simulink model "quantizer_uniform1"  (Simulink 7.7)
settings: Solver=FixedStepDiscrete  StartTime=0.0  StopTime=10  FixedStep=1/fs  RelTol=1e-3
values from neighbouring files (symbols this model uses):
  k = sqrt(10^(atenuation/10))    [quantizer_test.m]
undefined symbols (not defined in the file or in its folder): fs
libraries: dspquant2 x1, dspsrcs4 x1

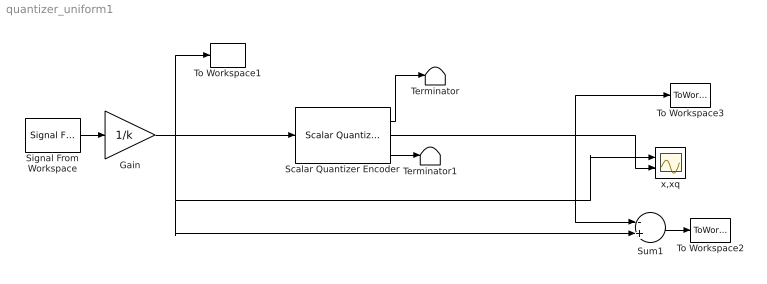
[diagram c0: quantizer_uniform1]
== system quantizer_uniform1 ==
  Gain : Gain  Gain=1/k
  Scalar Quantizer Encoder : dspquant2/Scalar Quantizer Encoder  paramSrc=Specify via dialog  partType=Bounded  BBoundary=boundary  UBoundary=[2:9]  SearchMethod=Linear  tieBreakRule=Choose the lower index  outQU=on  outQError=on  codebook=codebook  outStatus=off  invalidin=Clip  idtype=int32  roundingMode=Floor  overflowMode=off
  Signal From Workspace : dspsrcs4/Signal From Workspace  SystemSampleTime=-1  X=x  Ts=1/fs  nsamps=1  OutputAfterFinalValue=Setting to zero  ignoreOrWarnInputAndFrameLengths=off
  Sum1 : Sum  Inputs=-+
  Terminator : Terminator
  Terminator1 : Terminator
  To Workspace1 : ToWorkspace  VariableName=xout  SampleTime=-1  SaveFormat=Array
  To Workspace2 : ToWorkspace  VariableName=eq  SampleTime=-1  SaveFormat=Array
  To Workspace3 : ToWorkspace  VariableName=xq  SampleTime=-1  SaveFormat=Array
  x,xq : Scope  NumInputPorts=2
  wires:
  Signal From Workspace/1 -> Gain/1
  Scalar Quantizer Encoder/2 -> Sum1/1, To Workspace3/1, x,xq/2
  Scalar Quantizer Encoder/1 -> Terminator/1
  Scalar Quantizer Encoder/3 -> Terminator1/1
  Gain/1 -> To Workspace1/1, Sum1/2, x,xq/1, Scalar Quantizer Encoder/1
  Sum1/1 -> To Workspace2/1
